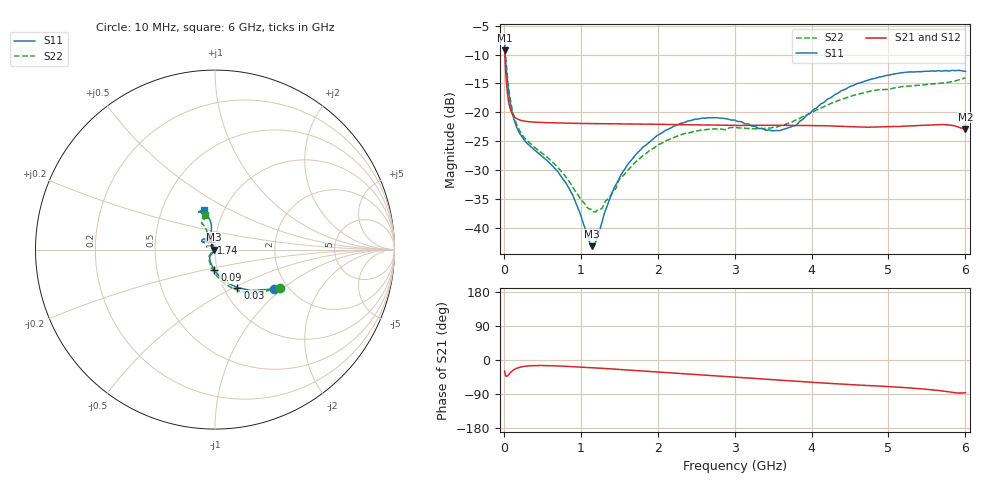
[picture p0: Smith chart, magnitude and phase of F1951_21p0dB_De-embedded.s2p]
! Integrated Device Technology
! Corporate Headquarters
! 6024 Silver Creek Valley Road
! San Jose, CA 95138  USA
! Phone:  1-408-284-8200
! Toll Free:  1-800-223-1366
! Webpage:  http://www.idt.com/
! Timing and RF Division
! 515 Groton Road, Suite 102
! Westford, MA 01886-6024
! Device:  F1951
! Description: 6-bit 0.5 dB Digital Step Attenuator
! Frequency:  100.0 -  4000.00 MHz
! Package:  4x4 mm Thin QFN Plastic Package: 24 pin
! Ports:  2 RF, 6 DC
!  Pin  1  = NC
!  Pin  2  = RF1  =  Port 1
!  Pin  3  = GND
!  Pin  4  = NC
!  Pin  5  = Serial Data Out (SDO)
!  Pin  6  = NC
!  Pin  7  = Reset Bar ( RSTb)
!  Pin  8  = Clock (CLK)
!  Pin  9  = Chip Select Bar (CSb)
!  Pin 10  = NC
!  Pin 11  = Serial Data In (SDI)
!  Pin 12  = NC
!  Pin 13  = NC
!  Pin 14  = VDD
!  Pin 15  = NC
!  Pin 16  = GND
!  Pin 17  = RF2  =  Port 2
!  Pin 18  = NC
!  Pin 19  = GND
!  Pin 20  = GND
!  Pin 21  = GND
!  Pin 22  = GND
!  Pin 23  = GND
!  Pin 24  = GND
! State:  42
! Atten State:  21.0 dB
! Voltage:  +3.30 Volts
! Current:  0.479 mA
! Data:  The device was measured on a F195X evaluation board which has
!  individual transmission lines to the RF pins.  Data was collected
!  de-embedded using a Automatic Fixture Removal [AFR] (Keysight Technologies).
!  The reference plane is the edge of the package pin.
! Misc:  Lot Code  1225BCA
!  Action Tracker AT0399
! Date Measured:  2018-09-13
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# GHz S dB R 50
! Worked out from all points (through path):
!   600 points, 10 MHz to 6 GHz, reference 50 ohm
!   highest |S21| = -9.26 dB at 10 MHz (marker M1); lowest = -22.9 dB at 6 GHz (marker M2)
!   group delay of S21, straight-line fit = 33.9 ps
!   lowest |S11| = -43.2 dB at 1.15 GHz (marker M3), VSWR 1.01, Z = 49.3 + j0.0441 ohm
!   |S11| at or under -10 dB: 18.43 MHz to end of sweep
!   |S22| runs from -37.3 to -7.6 dB; largest |S21 - S12| = 0.00023
!   S11 on the Smith chart (normalised r, x): 10 MHz: 1.70, -0.88; 30 MHz: 1.16, -0.52; 90 MHz: 0.97, -0.22; 1.74 GHz: 0.96, +0.08; 6 GHz: 0.81, +0.37
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0.01  -8.02 -33.5  -9.26 -29.4  -9.26 -29.4  -7.55 -30.8
0.03  -12.20 -59.4  -14.09 -43.0  -14.09 -43.1  -11.43 -59.5
0.06  -16.19 -79.5  -18.01 -39.3  -18.02 -39.3  -15.58 -80.9
0.09  -18.85 -91.5  -19.70 -32.3  -19.70 -32.2  -18.29 -93.4
0.16  -22.35 -108.5  -21.03 -22.4  -21.03 -22.4  -21.89 -110.5
0.25  -24.53 -119.3  -21.49 -17.3  -21.49 -17.2  -24.13 -122.1
0.72  -30.62 -126.3  -21.85 -15.9  -21.85 -15.9  -29.85 -136.5
0.88  -33.98 -128.0  -21.90 -17.5  -21.89 -17.5  -32.61 -141.0
1.01  -38.30 -136.5  -21.94 -18.9  -21.94 -18.8  -35.26 -149.8
1.15  -43.20 176.3  -21.95 -20.3  -21.95 -20.3  -36.98 -172.3
1.27  -39.33 127.0  -21.96 -21.8  -21.96 -21.8  -36.70 162.2
1.44  -32.96 113.9  -21.99 -24.1  -21.99 -24.1  -33.41 141.1
1.74  -26.99 116.2  -22.02 -28.1  -22.03 -28.1  -28.33 131.7
2.01  -23.90 123.8  -22.08 -31.9  -22.08 -31.8  -25.61 134.1
2.49  -21.18 137.7  -22.18 -38.5  -22.17 -38.5  -23.27 141.8
3.01  -21.40 148.2  -22.27 -45.5  -22.27 -45.4  -22.61 145.4
3.58  -23.18 126.8  -22.25 -53.0  -22.25 -53.1  -22.37 128.0
3.79  -22.29 110.7  -22.30 -55.9  -22.31 -55.9  -21.38 121.0
4.01  -19.74 101.7  -22.30 -58.9  -22.30 -58.9  -20.01 115.6
4.49  -15.59 99.4  -22.49 -65.1  -22.49 -65.1  -17.30 114.0
5.01  -13.56 108.0  -22.50 -70.1  -22.50 -70.1  -16.02 116.6
6  -12.88 105.8  -22.90 -86.4  -22.90 -86.4  -14.02 105.7
